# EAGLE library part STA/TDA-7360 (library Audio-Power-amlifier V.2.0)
20W BRIDGE/STEREO AUDIO AMPLIFIER WITH CLIPPING DETECTOR
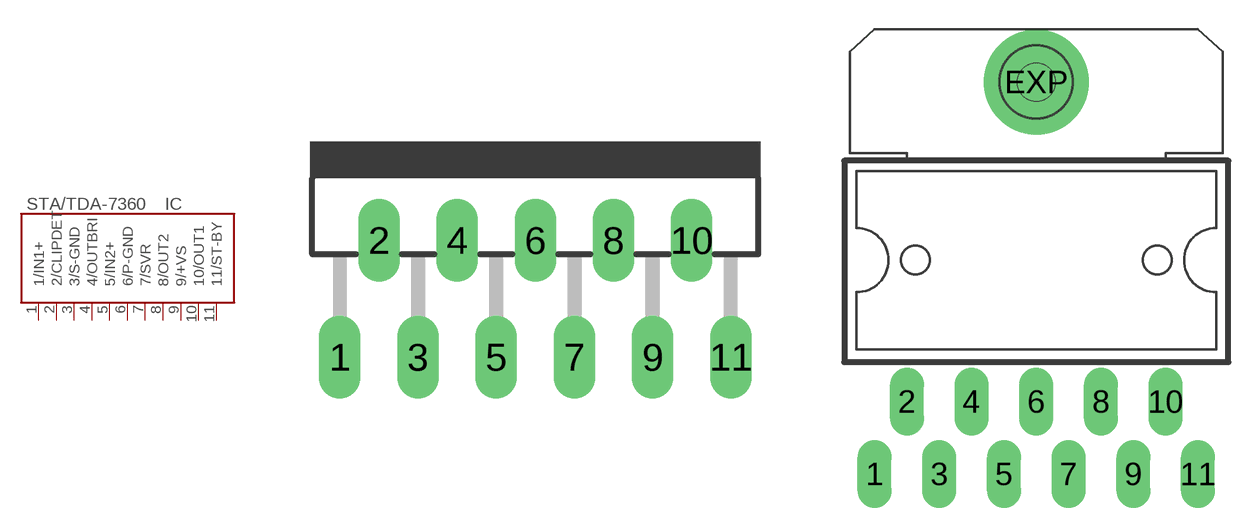
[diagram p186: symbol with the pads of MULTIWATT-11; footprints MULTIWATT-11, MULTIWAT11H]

Designator prefix IC

## STA/TDA-7360TDA7360/STA7360  [MULTIWATT-11]
1  1/IN1+  in
2  2/CLIPDET
3  3/S-GND  pwr
4  4/OUTBRI  out
5  5/IN2+  in
6  6/P-GND  pwr
7  7/SVR
8  8/OUT2  out
9  9/+VS  pwr
10  10/OUT1  out
11  11/ST-BY  in

## STA/TDA-7360TDA7360_ONLY  [MULTIWAT11H]
Pads as for MULTIWATT-11

## Footprint MULTIWATT-11 (pad centres in mm)
Muliwatt 11 lead
drill 1.2 long: 1 -8.5,-6.35; 2 -6.8,-1.27; 3 -5.1,-6.35; 4 -3.4,-1.27; 5 -1.7,-6.35; 6 0,-1.27; 7 1.7,-6.35; 8 3.4,-1.27; 9 5.1,-6.35; 10 6.8,-1.27; 11 8.5,-6.35

## Footprint MULTIWAT11H (pad centres in mm)
Multiwatt11 H (Short leads)
drill 0.9 pad 1.778 long: 1 -8.5,-3.81; 2 -6.8,0; 3 -5.1,-3.81; 4 -3.4,0; 5 -1.7,-3.81; 6 0,0; 7 1.7,-3.81; 8 3.4,0; 9 5.1,-3.81; 10 6.8,0; 11 8.5,-3.81
drill 3.2 pad 5.5: EXP 0,16.81
hole 2 at 0,16.81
